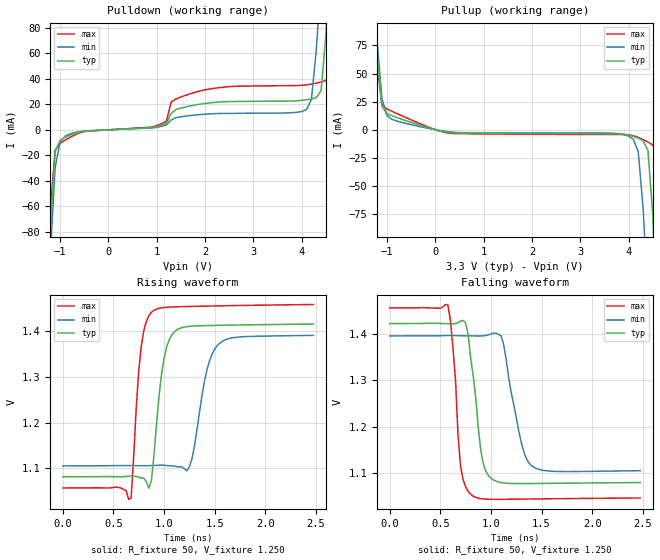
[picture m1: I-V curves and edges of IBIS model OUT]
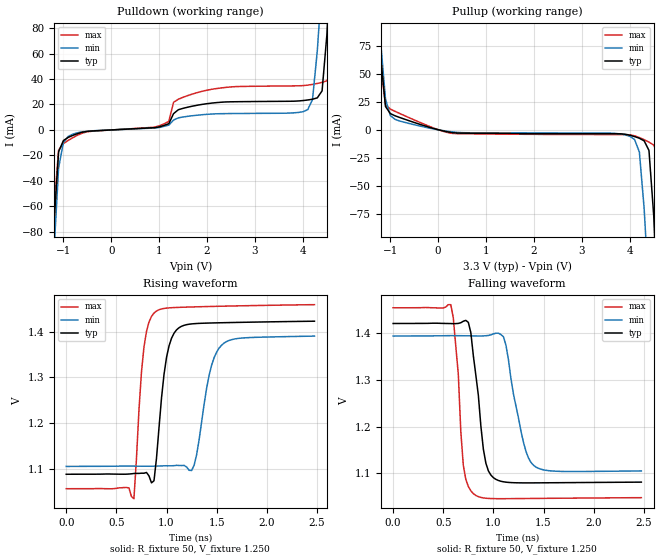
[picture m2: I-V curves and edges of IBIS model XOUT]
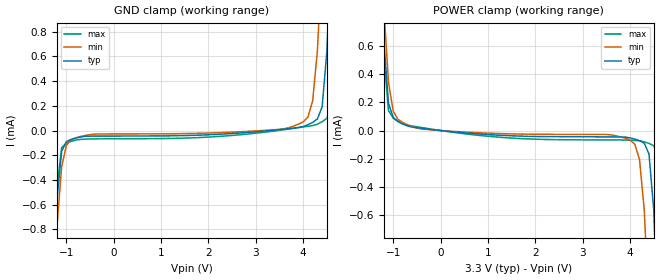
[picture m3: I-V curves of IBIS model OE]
[IBIS Ver]   3.2
[Comment Char]   |_char
[File name]   vg5032vdn.ibs
[File Rev]   1.0
[Date]   2015/07/30 5:46:34
[Source]
[Notes]
[Disclaimer]
Seiko Epson Corporation makes no warranty with respect to the information
contained herein.
[Copyright]
Copyright(C) 2014, Seiko Epson Corporation. All rights reserved.
[Component]   vg5032vdn
Si_location Pin
Timing_location Pin
[Manufacturer]   Seiko Epson Corporation
[Package]
R_pkg   0.36   NA   NA
L_pkg   4.00n   NA   NA
C_pkg   0.42p   NA   NA
[Pin] signal_name   model_name   R_pin   L_pin   C_pin
1   VC   NC
2   OE   OE   0.10   2.00n   0.77p
3   GND   GND
4   OUT   OUT   0.43   4.00n   0.47p
5   XOUT   XOUT   0.28   4.00n   0.38p
6   VCC   POWER
[Diff Pin] inv_pin vdiff   tdelay_typ
4   5   0   0
| Models and submodels in the file (3): OUT (Output), XOUT (Output), OE (Input)
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[Model]   OUT
Model_type Output
Enable Active-High
Polarity Non-Inverting
Vref=1.250
Vmeas=1.250
Rref=50
Cref=0
C_comp   0.1p   0.1p   0.1p
[Temperature Range] 25   105   -40
[Voltage Range]   3.3   3.135   3.465
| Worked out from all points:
|   slope of the pulldown table from 0 to 0.495 V, typ, clamps not added: 504 ohm
|   slope of the pullup table from 0 to 0.495 V, typ, clamps not added: 162 ohm
|   falling waveform, R_fixture 50, V_fixture 1.250: 20-80 % time 103ps typ, 148ps min, 71.7ps max; typ from 1.42 V to 1.08 V
|   rising waveform, R_fixture 50, V_fixture 1.250: 20-80 % time 100ps typ, 138ps min, 80.2ps max; typ from 1.08 V to 1.42 V
[Pullup]
-3.3V     1.626A     1.26A      2.031A
-1.3V     139.3mA    134.1mA    152mA
-1.2V     65.25mA    78.11mA    58.27mA
-1.1V     20.87mA    27.61mA    22.31mA
-800mV    11mA       7.847mA    14.57mA
4V        -4.789mA   -5.715mA   -4.464mA
4.2V      -7.52mA    -19.83mA   -6.897mA
4.4V      -18.39mA   -147.3mA   -10.96mA
4.5V      -76.97mA   -224.2mA   -13.67mA
4.6V      -179mA     -301.2mA   -23.37mA
4.7V      -281.2mA   -378.3mA   -110.2mA
6.6V      -2.221A    -1.843A    -2.564A
[Pulldown]
-3.3V     -2.257A    -1.744A    -2.818A
-1.3V     -179.6mA   -176.6mA   -193.2mA
-1.2V     -76.33mA   -98.31mA   -63.45mA
-1.1V     -17.19mA   -29.84mA   -15.98mA
-800mV    -4.312mA   -3.344mA   -6.091mA
4V        23.03mA    14.22mA    34.79mA
4.2V      24.08mA    23.75mA    35.76mA
4.4V      30.68mA    117.4mA    37.38mA
4.5V      74.68mA    172.8mA    38.62mA
4.6V      148.1mA    228.2mA    44.86mA
4.7V      221.5mA    283.7mA    109.4mA
6.6V      1.633A     1.352A     1.896A
[Falling Waveform]
R_fixture=50
V_fixture=1.250
V_fixture_min=1.250
V_fixture_max=1.250
0s        1.421V     1.395V     1.455V
575ps     1.421V     1.396V     1.461V
650ps     1.421V     1.395V     1.301V
700ps     1.426V     1.395V     1.116V
800ps     1.347V     1.395V     1.055V
900ps     1.149V     1.395V     1.046V
1ns       1.09V      1.399V     1.044V
1.1ns     1.08V      1.395V     1.044V
1.4ns     1.078V     1.117V     1.045V
2.475ns   1.08V      1.106V     1.047V
[Rising Waveform]
R_fixture=50
V_fixture=1.250
V_fixture_min=1.25
V_fixture_max=1.25
0s        1.081V     1.105V     1.057V
675ps     1.083V     1.106V     1.034V
775ps     1.078V     1.106V     1.368V
900ps     1.127V     1.106V     1.446V
1ns       1.341V     1.106V     1.453V
1.1ns     1.399V     1.105V     1.454V
1.25ns    1.411V     1.103V     1.455V
1.425ns   1.413V     1.317V     1.456V
1.55ns    1.413V     1.374V     1.456V
2.475ns   1.416V     1.391V     1.459V
[Ramp]
R_load=50
dV/dt_r   2.028e-1/1.021e-10   2.442e-1/1.473e-10   2.430e-1/8.101e-11
dV/dt_f   2.028e-1/1.018e-10   2.442e-1/1.357e-10   2.430e-1/6.919e-11
|[End   OUT
[Model]   XOUT
Model_type Output
Enable Active-High
Polarity Inverting
Vref=1.250
Vmeas=1.250
Rref=50
Cref=0
C_comp   0.1p   0.1p   0.1p
[Temperature Range] 25   105   -40
[Voltage Range]   3.3   3.135   3.465
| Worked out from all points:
|   slope of the pulldown table from 0 to 0.495 V, typ, clamps not added: 504 ohm
|   slope of the pullup table from 0 to 0.495 V, typ, clamps not added: 162 ohm
|   falling waveform, R_fixture 50, V_fixture 1.250: 20-80 % time 103ps typ, 150ps min, 71.3ps max; typ from 1.42 V to 1.08 V
|   rising waveform, R_fixture 50, V_fixture 1.250: 20-80 % time 100ps typ, 136ps min, 80.3ps max; typ from 1.09 V to 1.42 V
[Pullup]
-3.3V     1.626A     1.26A      2.031A
-1.3V     139.3mA    134.1mA    152mA
-1.2V     65.25mA    78.11mA    58.27mA
-1.1V     20.87mA    27.61mA    22.31mA
-800mV    11mA       7.847mA    14.57mA
4V        -4.789mA   -5.715mA   -4.464mA
4.2V      -7.52mA    -19.83mA   -6.897mA
4.4V      -18.39mA   -147.3mA   -10.96mA
4.5V      -76.97mA   -224.2mA   -13.67mA
4.6V      -179mA     -301.2mA   -23.37mA
4.7V      -281.2mA   -378.3mA   -110.2mA
6.6V      -2.221A    -1.843A    -2.564A
[Pulldown]
-3.3V     -2.257A    -1.744A    -2.818A
-1.3V     -179.6mA   -176.6mA   -193.2mA
-1.2V     -76.33mA   -98.31mA   -63.45mA
-1.1V     -17.19mA   -29.84mA   -15.98mA
-800mV    -4.312mA   -3.344mA   -6.091mA
4V        23.03mA    14.22mA    34.79mA
4.2V      24.08mA    23.75mA    35.76mA
4.4V      30.68mA    117.4mA    37.38mA
4.5V      74.68mA    172.8mA    38.62mA
4.6V      148.1mA    228.2mA    44.86mA
4.7V      221.5mA    283.7mA    109.4mA
6.6V      1.633A     1.352A     1.896A
[Falling Waveform]
R_fixture=50
V_fixture=1.250
V_fixture_min=1.250
V_fixture_max=1.250
0s        1.421V     1.394V     1.455V
575ps     1.421V     1.395V     1.462V
650ps     1.421V     1.395V     1.313V
700ps     1.426V     1.395V     1.117V
800ps     1.352V     1.395V     1.056V
900ps     1.152V     1.395V     1.047V
1ns       1.091V     1.399V     1.046V
1.1ns     1.082V     1.393V     1.046V
1.4ns     1.079V     1.117V     1.046V
2.475ns   1.081V     1.105V     1.048V
[Rising Waveform]
R_fixture=50
V_fixture=1.250
V_fixture_min=1.250
V_fixture_max=1.250
0s        1.088V     1.105V     1.057V
675ps     1.09V      1.106V     1.035V
775ps     1.091V     1.106V     1.366V
900ps     1.123V     1.106V     1.445V
1ns       1.344V     1.107V     1.451V
1.1ns     1.404V     1.108V     1.453V
1.275ns   1.417V     1.108V     1.454V
1.425ns   1.419V     1.305V     1.455V
1.55ns    1.419V     1.37V      1.455V
2.475ns   1.423V     1.39V      1.459V
[Ramp]
R_load=50
dV/dt_r   2.028E-1/1.020E-10   2.442E-1/1.476E-10   2.430E-1/8.126E-11
dV/dt_f   2.028E-1/1.011E-10   2.442E-1/1.395E-10   2.430E-1/6.914E-11
|[End   XOUT
[Model]   OE
Model_type Input
Vinh=2.31
Vinl=0.99
C_comp   2p   2p   2p
[Temperature Range] 25   105   -40
[Voltage Range]   3.3   3.135   3.465
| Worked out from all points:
|   GND clamp passes 1 mA (typ) near -1.25 V on its own axis
|   POWER clamp passes 1 mA (typ) near -1.24 V on its own axis
[GND Clamp]
-3.3V     -24.59mA   -20.62mA   -29.61mA
-1.3V     -1.492mA   -1.611mA   -1.557mA
-1.2V     -564.6uA   -781.1uA   -469.2uA
-1.1V     -167.5uA   -293.8uA   -139.5uA
-900mV    -71.67uA   -74.5uA    -87.5uA
4V        32.36uA    70.23uA    28.73uA
4.2V      65.85uA    240.3uA    40.14uA
4.3V      93.27uA    645.4uA    51.34uA
4.4V      191.4uA    1.414mA    71.39uA
4.6V      1.622mA    3.388mA    204.2uA
4.7V      2.825mA    4.381mA    851.7uA
6.6V      25.83mA    23.34mA    28.68mA
[POWER Clamp]
-3.3V     25.83mA    21.69mA    31.12mA
-1.3V     1.622mA    1.749mA    1.684mA
-1.2V     640.5uA    876.4uA    526.2uA
-1.1V     191.4uA    340.9uA    141.8uA
-1V       93.27uA    137uA      87.41uA
-700mV    32.36uA    41.55uA    37.98uA
4V        -52.14uA   -67.57uA   -68.59uA
4.2V      -71.67uA   -206.7uA   -72.81uA
4.4V      -167.5uA   -1.289mA   -91.72uA
4.6V      -1.492mA   -3.174mA   -189.7uA
4.7V      -2.641mA   -4.121mA   -767.5uA
6.6V      -24.59mA   -22.2mA    -27.29mA
